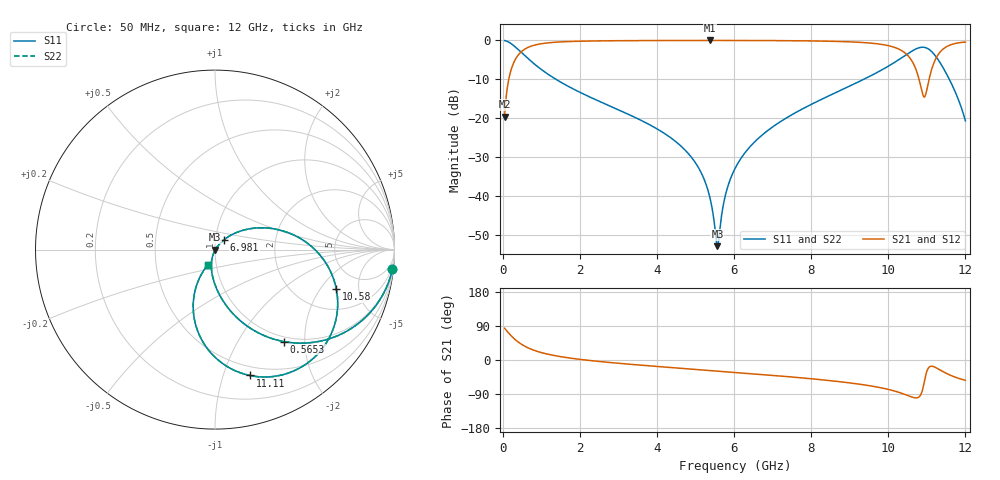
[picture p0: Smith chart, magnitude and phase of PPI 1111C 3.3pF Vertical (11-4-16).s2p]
# GHz S MA R 50
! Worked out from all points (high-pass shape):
!   1601 points, 50 MHz to 12 GHz, reference 50 ohm
!   highest |S21| = -0.02 dB at 5.368 GHz (marker M1); lowest = -19.6 dB at 50 MHz (marker M2)
!   |S21| within 3 dB of the highest: 472.5 MHz to 10.41 GHz (9.934 GHz wide, 183 % of centre); 11.34 GHz to end of sweep
!   lowest |S11| = -53.0 dB at 5.569 GHz (marker M3), VSWR 1.00, Z = 50.2 - j0.113 ohm
!   |S11| at or under -10 dB: 1.378 GHz to 9.369 GHz (7.991 GHz wide, 149 % of centre); 11.58 GHz to end of sweep
!   |S22| runs from -53.0 to 0.0 dB; largest |S21 - S12| = 0
!   S11 on the Smith chart (normalised r, x): 50 MHz: 1, -18; 565.3 MHz: 0.92, -1.60; 6.981 GHz: 1.10, +0.12; 10.58 GHz: 3.22, -2.87; 11.11 GHz: 0.41, -1.23; 12 GHz: 0.91, -0.15
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0.05  0.9945 -6.3  0.1047 83.7  0.1047 83.7  0.9945 -6.3
0.1545625  0.9508 -18.9  0.3095 71.1  0.3095 71.1  0.9508 -18.9
0.2441875  0.8891 -28.5  0.4574 61.4  0.4574 61.4  0.8891 -28.5
0.5653438  0.6411 -53.1  0.7669 36.8  0.7669 36.8  0.6411 -53.1
1.095625  0.3907 -72.8  0.9196 17.1  0.9196 17.1  0.3907 -72.8
2.044156  0.2097 -88.5  0.9764 1.2  0.9764 1.2  0.2097 -88.5
4.038312  0.07088 -105.9  0.9955 -17.3  0.9955 -17.3  0.07088 -105.9
4.919625  0.03016 -110.4  0.9973 -24.2  0.9973 -24.2  0.03016 -110.4
5.1885  0.01794 -109.5  0.9974 -26.2  0.9974 -26.2  0.01794 -109.5
5.36775  0.009765 -104.8  0.9975 -27.6  0.9975 -27.6  0.009765 -104.8
5.569406  0.002244 -30.2  0.9974 -29.1  0.9974 -29.1  0.002244 -30.2
5.786  0.01064 46.5  0.9973 -30.8  0.9973 -30.8  0.01064 46.5
6.025  0.02239 51.0  0.997 -32.7  0.997 -32.7  0.02239 51.0
6.981  0.07565 47.3  0.9937 -40.4  0.9937 -40.4  0.07565 47.3
8.019156  0.1515 38.6  0.9836 -49.7  0.9836 -49.7  0.1515 38.6
10.01331  0.4692 8.4  0.8525 -77.9  0.8525 -77.9  0.4692 8.4
10.58094  0.7112 -18.1  0.575 -96.6  0.575 -96.6  0.7112 -18.1
10.76766  0.7946 -34.3  0.3572 -99.3  0.3572 -99.3  0.7946 -34.3
10.9245  0.8146 -51.8  0.1876 -62.7  0.1876 -62.7  0.8146 -51.8
11.11122  0.7279 -74.5  0.4005 -16.5  0.4005 -16.5  0.7279 -74.5
11.43984  0.4286 -104.7  0.7858 -31.8  0.7858 -31.8  0.4286 -104.7
12  0.09213 -115.1  0.9521 -53.7  0.9521 -53.7  0.09213 -115.1
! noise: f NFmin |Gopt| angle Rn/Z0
0.05  0.0004971  0.9183  2.767  0.001343
1.372  0.003725  0.6733  8.888  0.002184
2.701  0.006048  0.6193  15.43  0.002911
4.031  0.00821  0.5942  21.91  0.003588
5.36  0.01047  0.5877  28.18  0.004387
6.682  0.01323  0.6007  34.16  0.005613
8.012  0.01779  0.6455  40.06  0.008441
9.341  0.03059  0.7531  46.21  0.02123
10.67  0.1879  0.9508  52.67  0.689
12  0.06442  0.8525  58.37  0.07114
